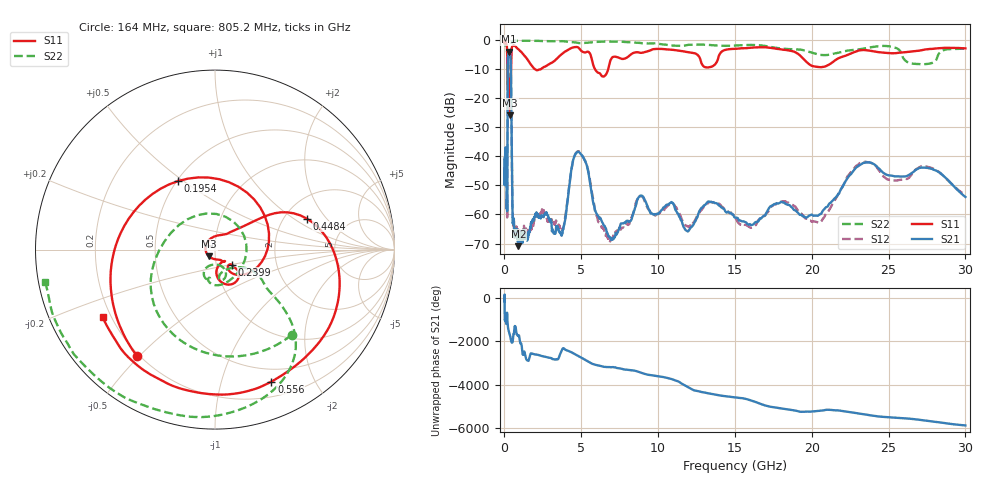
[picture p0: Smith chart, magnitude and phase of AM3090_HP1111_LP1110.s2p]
! Date/Time: Thu, Feb 28, 2019 2:10 PM
! Network Analyzer: Agilent Technologies E8364B Rev: A.07.50.67
! Sweep from 0.010 to 30.000 GHz, 1601 Points, Sweep Type: LOG
! Power Supply: 5.023 V, 0.002 A
# Hz S DB R 50
!freq MagS11 AngS11 MagS21 AngS21 MagS12 AngS12 MagS22 AngS22
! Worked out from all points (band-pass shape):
!   1601 points, 10 MHz to 30 GHz, reference 50 ohm
!   highest |S21| = -4.05 dB at 290.1 MHz (marker M1); lowest = -70.9 dB at 903.4 MHz (marker M2)
!   |S21| within 3 dB of the highest: 222.2 MHz to 403.8 MHz (181.6 MHz wide, 58 % of centre)
!   lowest |S11| = -25.9 dB at 378.2 MHz (marker M3), VSWR 1.11, Z = 46.6 - j3.54 ohm
!   |S11| at or under -10 dB: 207.3 MHz to 430.6 MHz (223.3 MHz wide, 70 % of centre); 1.972 GHz to 2.384 GHz (411.1 MHz wide, 18.9 % of centre); 5.884 GHz to 6.755 GHz (870.1 MHz wide, 13.8 % of centre)
!   |S22| runs from -21.6 to -0.2 dB; largest |S21 - S12| = 0.013
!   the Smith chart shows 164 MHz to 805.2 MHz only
!   S11 on the Smith chart (normalised r, x): 164 MHz: 0.19, -0.49; 195.4 MHz: 0.51, +0.48; 239.9 MHz: 1.19, -0.20; 448.4 MHz: 2.65, +1.29; 556 MHz: 0.36, -1.46; 805.2 MHz: 0.17, -0.27
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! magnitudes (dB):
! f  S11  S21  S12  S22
! 10 MHz  -0.3  -40.8  -47.2  -0.7
! 38.04 MHz  -0.3  -41.1  -40.8  -1.4
! 102.5 MHz  -0.9  -39.4  -38.9  -2.9
! 144.7 MHz  -1.7  -55.2  -55.5  -3.6
! 164 MHz  -2.7  -55.5  -56.4  -3.9
! 181.3 MHz  -4.5  -56.9  -59.5  -5.1
! 195.4 MHz  -7.3  -36.1  -36.4  -10.9
! 212.7 MHz  -11.8  -10.8  -10.8  -14.4
! 239.9 MHz  -18.1  -5.0  -5.0  -15.6
! 290.1 MHz  -13.8  -4.1  -4.0  -20.7
! 378.2 MHz  -25.9  -5.2  -5.2  -15.6
! 448.4 MHz  -5.3  -24.0  -24.0  -2.1
! 550.5 MHz  -2.0  -62.5  -61.6  -0.4
! 556 MHz  -1.9  -63.0  -63.1  -0.4
! 805.2 MHz  -2.7  -66.7  -64.7  -0.3
! 903.4 MHz  -3.2  -70.9  -66.0  -0.3
! 2.084 GHz  -10.4  -59.3  -60.6  -0.3
! 3.723 GHz  -4.9  -67.3  -65.3  -0.4
! 4.805 GHz  -2.6  -38.5  -38.2  -1.1
! 6.653 GHz  -11.5  -66.2  -67.4  -0.6
! 7.926 GHz  -6.2  -62.3  -63.3  -0.7
! 30 GHz  -2.9  -54.0  -53.2  -3.0
